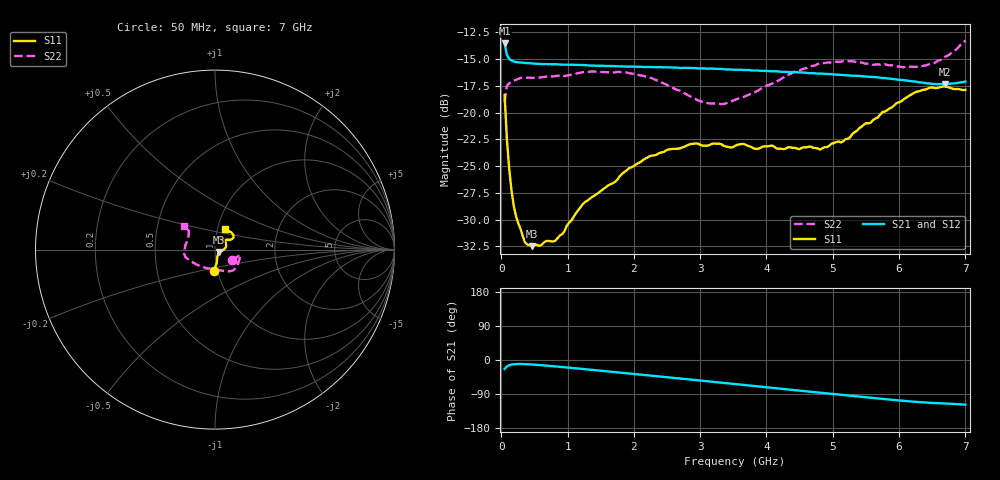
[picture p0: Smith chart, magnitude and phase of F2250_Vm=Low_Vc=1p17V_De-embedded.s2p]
! Integrated Device Technology
! Corporate Headquarters
! 6024 Silver Creek Valley Road
! San Jose, CA 95138  USA
! Phone:  1-408-284-8200
! Toll Free:  1-800-223-1366
! Webpage:  http://www.idt.com/
! Timing and RF Division
! 515 Groton Road, Suite 102
! Westford, MA 01886-6024
! Device:  F2250
! Description: Voltage Variable RF Attenuator
! Frequency:  50.0 -  6000.00 MHz
! Package:  3x3 mm Thin QFN Plastic Package: 16 pin
! Ports:  2 RF, 3 DC
!  Pin  1  = GND
!  Pin  2  = NC
!  Pin  3  = RF1  = Port 1
!  Pin  4  = NC
!  Pin  5  = GND
!  Pin  6  = GND
!  Pin  7  = GND
!  Pin  8  = GND
!  Pin  9  = NC
!  Pin 10  = RF2  = Port 2
!  Pin 11  = NC
!  Pin 12  = GND
!  Pin 13  = GND
!  Pin 14  = VCNTRL
!  Pin 15  = VDD
!  Pin 16  = VMODE
! Vcntrl:  1.170 Volts
! Vmode:  +0.000 Volts
! Vdd:  +3.30  Volts
! Current:  1.192 mA
! Data:  The device was measured on a the F2250 evaluation board which has
!  individual transmission lines to the RF pins.  Data was collected
!  using a calibrated network analyzer.  The evaluation board was
!  de-embedded using a TRL calibration technique.
!  The reference plane is the edge of the package pin.
! Misc:  SN 10
!  Action Tracker AT0258
! Date Measured:  2014-11-26
! Date:  2015-10-15  MJV
! Note:
!  Integrated Device Technology supplies this data as a sample of measured
!  data at the package pin for this product.  Your particular data for this
!  product may vary.
!  Data was taken at 25 degrees C.
!  Integrated Device Technology reserves the right to change this data at anytime.
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# GHz S dB R 50
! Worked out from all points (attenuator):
!   201 points, 50 MHz to 7 GHz, reference 50 ohm
!   highest |S21| = -13.54 dB at 50 MHz (marker M1); lowest = -17.4 dB at 6.687 GHz (marker M2)
!   lowest |S11| = -32.5 dB at 467 MHz (marker M3), VSWR 1.05, Z = 52 - j1.4 ohm
!   |S11| at or under -10 dB: start of sweep to end of sweep
!   |S22| runs from -19.2 to -13.3 dB; largest |S21 - S12| = 0.00065
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0.05  -18.36 -93.4  -13.54 -23.5  -13.55 -23.5  -18.99 -32.0
0.08475  -22.51 -82.6  -14.62 -17.0  -14.61 -17.0  -17.51 -16.5
0.1195  -25.27 -77.5  -14.99 -13.8  -14.97 -13.8  -17.26 -12.4
0.189  -28.75 -66.0  -15.23 -11.2  -15.24 -11.2  -17.01 -11.2
0.22375  -29.73 -59.5  -15.29 -10.7  -15.28 -10.7  -16.94 -11.7
0.36275  -32.18 -41.8  -15.37 -10.9  -15.38 -10.9  -16.76 -13.2
0.467  -32.48 -34.6  -15.42 -11.9  -15.42 -11.9  -16.76 -15.5
0.8145  -31.97 -18.2  -15.48 -16.9  -15.48 -16.9  -16.59 -25.8
1.2315  -28.54 -11.6  -15.56 -23.7  -15.56 -23.7  -16.23 -36.2
1.9265  -25.20 6.0  -15.70 -35.4  -15.69 -35.4  -16.31 -49.4
2.37825  -23.80 17.2  -15.76 -43.2  -15.77 -43.2  -17.04 -59.2
2.86475  -22.93 32.9  -15.84 -51.8  -15.83 -51.8  -18.54 -77.3
3.07325  -23.09 39.8  -15.88 -55.5  -15.87 -55.5  -19.08 -88.7
3.35125  -23.09 50.8  -15.94 -60.4  -15.95 -60.4  -19.20 -106.3
3.525  -23.11 54.7  -16.01 -63.5  -15.99 -63.5  -18.81 -117.2
4.7065  -23.30 64.2  -16.33 -84.5  -16.33 -84.5  -15.64 -163.5
4.81075  -23.46 60.5  -16.36 -86.3  -16.34 -86.4  -15.40 -165.5
5.1235  -22.79 50.8  -16.48 -91.9  -16.48 -91.9  -15.25 -172.2
5.85325  -19.62 32.3  -16.84 -104.3  -16.83 -104.3  -15.59 171.4
6.2355  -18.13 33.5  -17.09 -110.2  -17.10 -110.2  -15.73 158.7
6.68725  -17.55 45.8  -17.36 -114.8  -17.35 -114.8  -14.82 144.1
7  -17.89 63.8  -17.11 -118.0  -17.09 -118.1  -13.27 142.4
